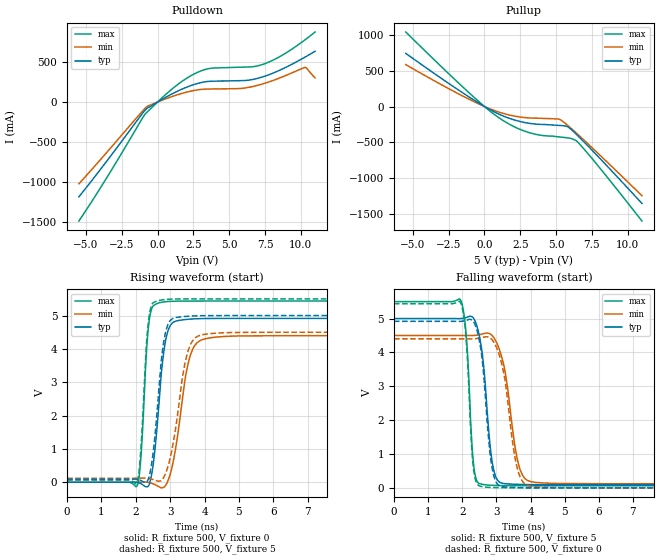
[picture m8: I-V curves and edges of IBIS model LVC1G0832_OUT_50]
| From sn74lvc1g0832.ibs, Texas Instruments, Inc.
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[Model]   LVC1G0832_OUT_50
Model_type  Output
Vref =   0
Rref =   500
Cref =   50p
Vmeas =   2.5
| variable   typ   min   max
C_comp   8.89pF   5.43pF   12.19pF
| C_pullup   9.59pF   5.43pF   12.19pF
| C_pulldown   8.19pF   6.18pF   11.58pF
[Temperature Range]   40   100   -40
| Ambient temperature   25   85   -40
[Voltage range]   5   4.5   5.5
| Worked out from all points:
|   slope of the pulldown table from 0 to 0.75 V, typ, clamps not added: 9.73 ohm
|   slope of the pullup table from 0 to 0.75 V, typ, clamps not added: 9.16 ohm
|   rising waveform, R_fixture 500, V_fixture 0: 20-80 % time 260ps typ, 377ps min, 171ps max; typ from 0 V to 4.91 V
|   falling waveform, R_fixture 500, V_fixture 5: 20-80 % time 256ps typ, 368ps min, 169ps max; typ from 5 V to 0.091 V
|   rising waveform, R_fixture 500, V_fixture 5: 20-80 % time 260ps typ, 388ps min, 172ps max; typ from 0.091 V to 5 V
|   falling waveform, R_fixture 500, V_fixture 0: 20-80 % time 253ps typ, 359ps min, 167ps max; typ from 4.92 V to 0 V
[Pulldown]
| LVC1G0832_OUT_50
|   Voltage   I(typ)   I(min)   I(max)
-5.5V     -1.19A     -1.026A    -1.493A
-3.615V   -756.5mA   -644.9mA   -968mA
-860mV    -99.61mA   -76.72mA   -149.6mA
1.155V    114.9mA    77.32mA    184.2mA
2.345V    207.1mA    137.1mA    331.4mA
3.395V    254.9mA    162mA      411.2mA
5.9V      268mA      171.6mA    436.9mA
6.79V     288mA      200mA      446mA
7.595V    330.4mA    241.1mA    487.6mA
8.825V    423.2mA    322.9mA    599.5mA
10.29V    561.5mA    432.7mA    778mA
11V       636.1mA    301.9mA    877.4mA
[Pullup]
| LVC1G0832_OUT_50
|   Voltage   I(typ)   I(min)   I(max)
-5.5V     745.2mA    587.5mA    1.044A
-1.18V    147.6mA    112.6mA    211.7mA
1.04V     -109.2mA   -79.97mA   -161.6mA
2.045V    -185.4mA   -131.8mA   -280mA
3.05V     -232.7mA   -158.7mA   -361.3mA
3.945V    -250.5mA   -165.3mA   -402.5mA
5.295V    -265.8mA   -184.8mA   -427.6mA
5.83V     -285.1mA   -267.5mA   -440mA
6.335V    -372.8mA   -357.2mA   -470.5mA
6.54V     -412.8mA   -394.7mA   -503.8mA
8.12V     -739mA     -692.4mA   -876.8mA
11V       -1.358A    -1.25A     -1.605A
[Ramp]
| LVC1G0832_OUT_50
| variable   typ   min   max
dV/dt_r   3.03/2.72E-10   2.74/4.00E-10   3.34/1.77E-10
dV/dt_f   2.98/2.65E-10   2.67/3.87E-10   3.31/1.78E-10
R_load = 500
[Rising Waveform]
| LVC1G0832_OUT_50
R_fixture =   500
C_fixture =   0
L_fixture =   0
V_fixture =   0
V_fixture_min = 0
V_fixture_max = 0
|   Time   V(typ)   V(min)   V(max)
0s        185.3pV    4.77nV     2.097nV
2.04ns    -3.734mV   317.3uV    -105mV
2.145ns   -42.27mV   2.084mV    709.1mV
2.31ns    -140mV     2.316mV    3.904V
2.405ns   -21.04mV   -15.42mV   4.957V
2.87ns    4.266V     -90.51mV   5.415V
3.105ns   4.809V     703mV      5.429V
3.605ns   4.894V     3.861V     5.434V
4.38ns    4.913V     4.358V     5.435V
50ns      4.914V     4.396V     5.435V
[Falling Waveform]
| LVC1G0832_OUT_50
R_fixture =   500
C_fixture =   0
L_fixture =   0
V_fixture =   5
V_fixture_min = 4.5
V_fixture_max = 5.5
|   Time   V(typ)   V(min)   V(max)
0s        5V         4.5V       5.5V
1.965ns   5V         4.5V       5.52V
2.12ns    5.031V     4.499V     4.461V
2.35ns    4.979V     4.5V       547.4mV
2.695ns   2.78V      4.568V     87.44mV
2.845ns   995mV      4.526V     75.84mV
3.005ns   275.1mV    4.292V     69.82mV
3.67ns    102.1mV    620.1mV    63.74mV
4.19ns    93.79mV    157.1mV    63.09mV
50ns      91.34mV    120.7mV    62.82mV
[Rising Waveform]
| LVC1G0832_OUT_50
R_fixture =   500
C_fixture =   0
L_fixture =   0
V_fixture =   5
V_fixture_min = 4.5
V_fixture_max = 5.5
|   Time   V(typ)   V(min)   V(max)
0s        91.33mV    120.7mV    62.82mV
2.035ns   89.08mV    121mV      -11.92mV
2.135ns   57.88mV    122.6mV    813.4mV
2.305ns   -7.258mV   123.6mV    4.066V
2.395ns   196.5mV    109.1mV    5.029V
2.85ns    4.42V      224.6mV    5.48V
3.07ns    4.91V      1.073V     5.494V
3.525ns   4.979V     3.949V     5.499V
4.21ns    4.998V     4.461V     5.5V
50ns      5V         4.5V       5.5V
[Falling Waveform]
| LVC1G0832_OUT_50
R_fixture =   500
C_fixture =   0
L_fixture =   0
V_fixture =   0
V_fixture_min = 0
V_fixture_max = 0
|   Time   V(typ)   V(min)   V(max)
0s        4.917V     4.401V     5.437V
1.96ns    4.917V     4.401V     5.454V
2.11ns    4.944V     4.399V     4.45V
2.34ns    4.893V     4.401V     492.1mV
2.675ns   2.74V      4.458V     22.66mV
2.83ns    895mV      4.418V     11.7mV
3ns       158.1mV    4.155V     6.102mV
3.62ns    9.921mV    553.9mV    947uV
4.105ns   2.475mV    34.12mV    304.1uV
50ns      12.97uV    19.52uV    7.332uV
